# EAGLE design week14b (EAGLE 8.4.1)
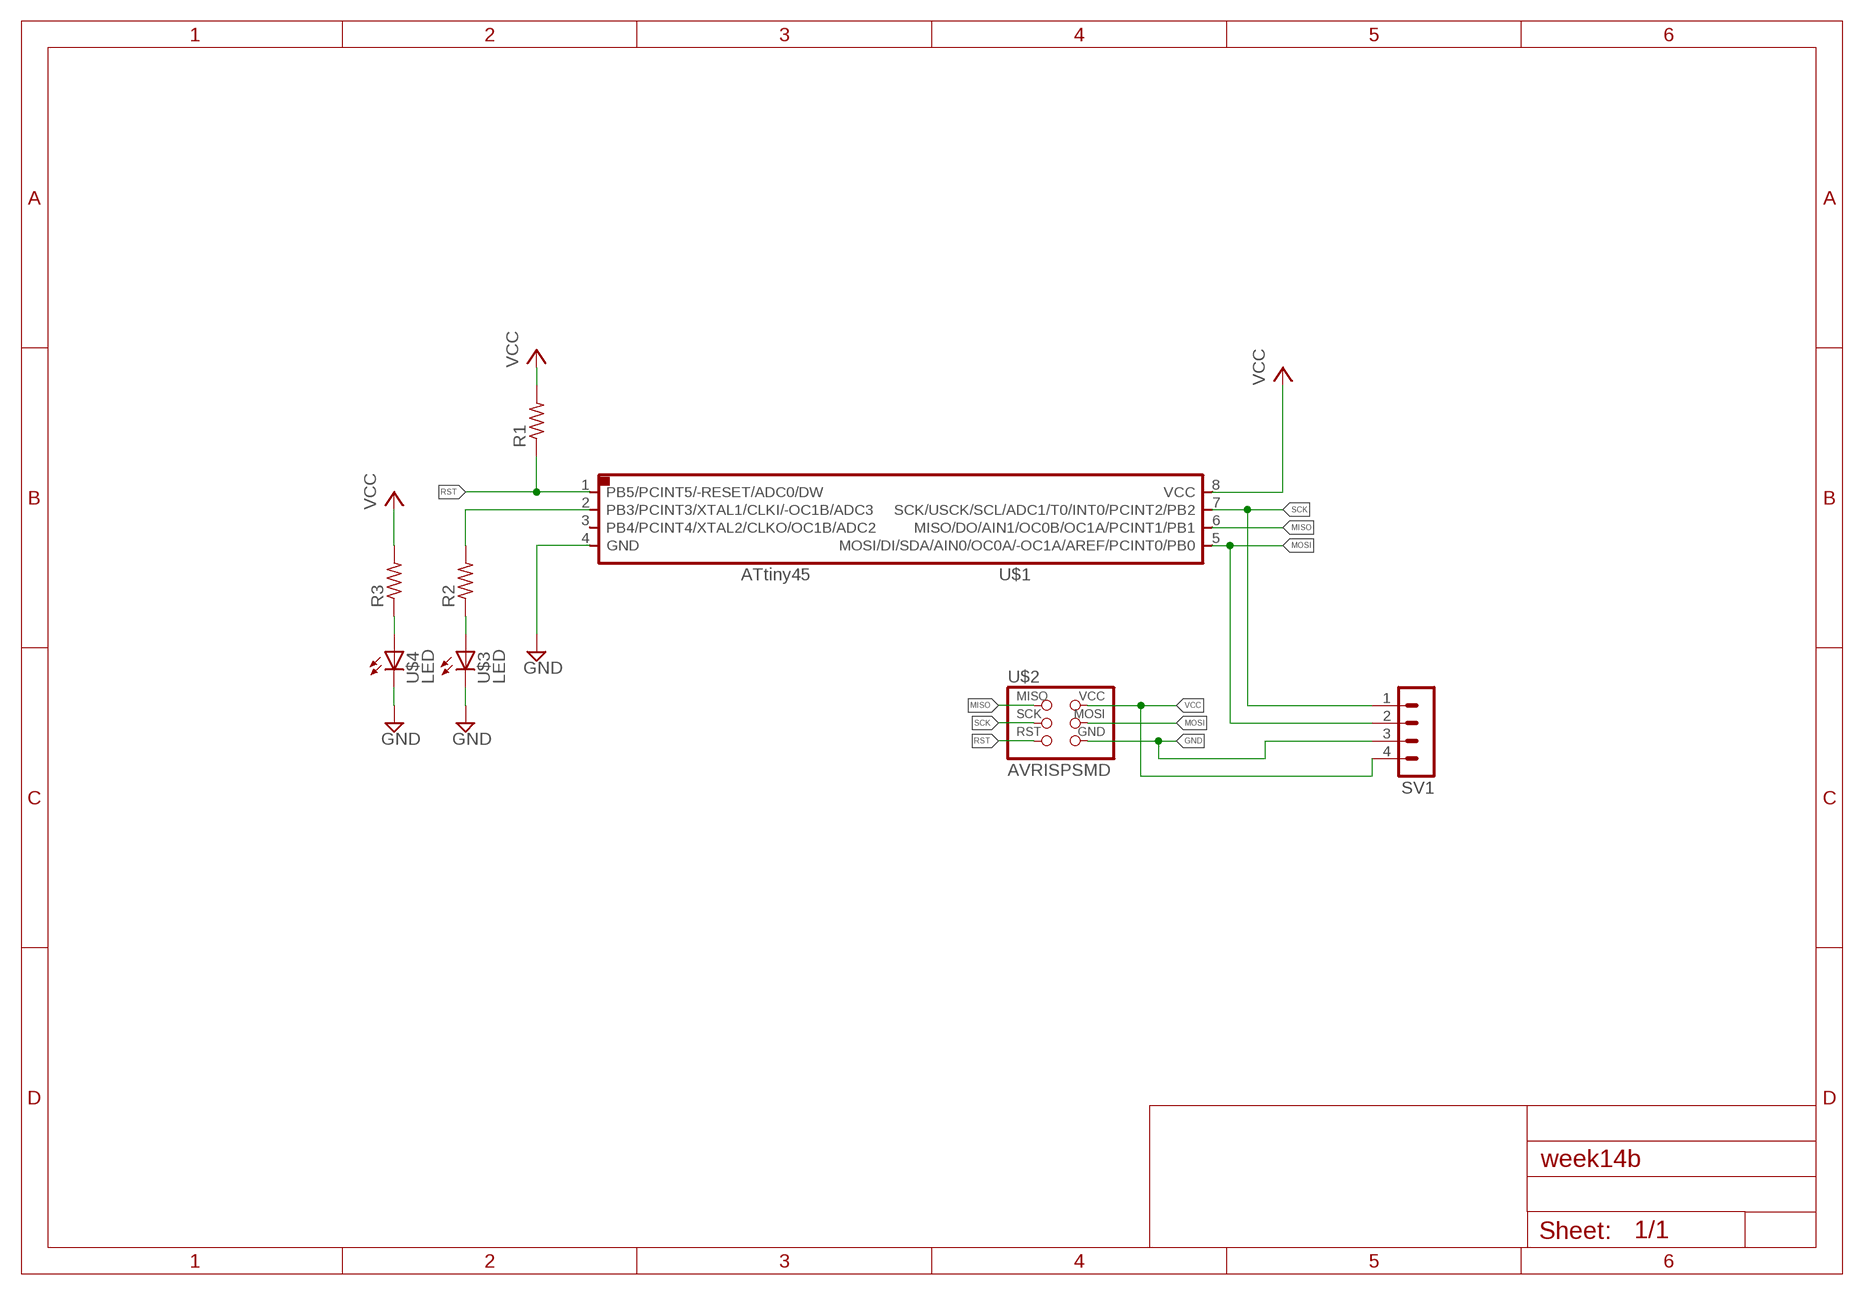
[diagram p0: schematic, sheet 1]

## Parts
R1  RES-US1206  [R1206]
R2  RES-US1206  [R1206]
R3  RES-US1206  [R1206]
SV1  MA04-1  [MA04-1]
U$1  ATTINY45SI  [SOIC8]
U$2  AVRISPSMD  [2X03SMD]
U$3  LED  [LED1206]
U$4  LED  [LED1206]

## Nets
GND: SV1.3 U$1.4(GND) U$2.6(GND) U$3.2(C) U$4.2(C)
MISO: U$1.6(MISO/DO/AIN1/OC0B/OC1A/PCINT1/PB1) U$2.1(MISO)
MOSI: SV1.2 U$1.5(MOSI/DI/SDA/AIN0/OC0A/-OC1A/AREF/PCINT0/PB0) U$2.4(MOSI)
N$2: R2.1 U$3.1(A)
N$3: R2.2 U$1.2(PB3/PCINT3/XTAL1/CLKI/-OC1B/ADC3)
N$5: R3.1 U$4.1(A)
RST: R1.1 U$1.1(PB5/PCINT5/-RESET/ADC0/DW) U$2.5(RST)
SCK: SV1.1 U$1.7(SCK/USCK/SCL/ADC1/T0/INT0/PCINT2/PB2) U$2.3(SCK)
VCC: R1.2 R3.2 SV1.4 U$1.8(VCC) U$2.2(VCC)
Unconnected: U$1.3(PB4/PCINT4/XTAL2/CLKO/OC1B/ADC2)

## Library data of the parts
R1-R3 = fab:RES-US: Resistor (US Symbol)
SV1 = con-lstb:MA04-1: PIN HEADER; OC_FARNELL: unknown; OC_NEWARK: unknown
U$1 = fab:ATTINY45
U$2 = fab:AVRISP
U$3 U$4 = fab:LED: LED

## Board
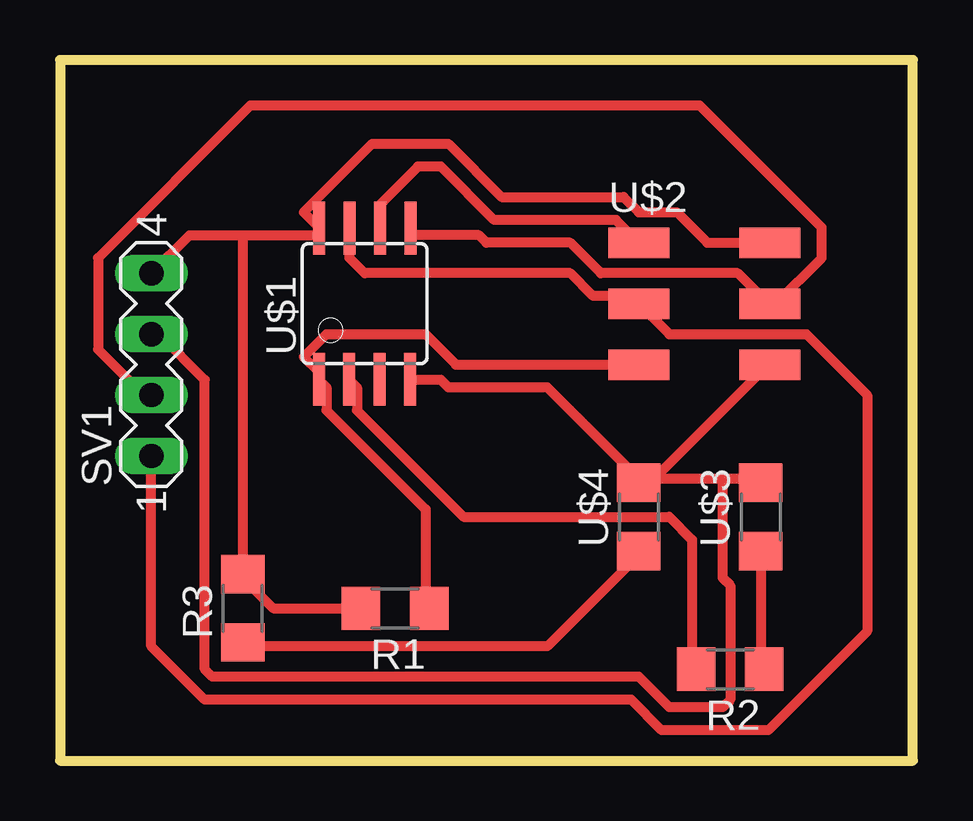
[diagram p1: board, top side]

Size 35.56 x 29.21 mm. Coordinates in mm from the lower left corner, seen from the top.
Outline: 0,29.21 0,0 35.56,0 35.56,29.21 0,29.21
Copper layers (1*16): Top 0.035mm / dielectric 1.5mm / Bottom 0.035mm
Design rules "default *": minimum track width 16mil, minimum drill 0.35mm, track to track 16mil, track to pad 16mil, pad to pad 16mil, via to via 6mil, smd to smd 16mil, copper to edge 16mil, drill to drill 16mil, minimum pad ring 10mil, minimum via ring 8mil, stop-mask expansion 4mil, vias tented up to drill 0mil, thermal gap 10mil

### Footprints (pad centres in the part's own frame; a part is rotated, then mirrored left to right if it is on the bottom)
R1206 = smd 1.6 x 1.803: 1 -1.422,0; 2 1.422,0
MA04-1 = drill 1.016 long: 1 -3.81,0; 2 -1.27,0; 3 1.27,0; 4 3.81,0
SOIC8 = smd 0.5 x 2.2: 1 -1.905,-3.154; 2 -0.645,-3.154; 3 0.625,-3.154; 4 1.895,-3.154; 5 1.905,3.154; 6 0.635,3.154; 7 -0.635,3.154; 8 -1.905,3.154
2X03SMD = smd 2.54 x 1.27: 1 -2.54,2.54; 2 2.92,2.54; 3 -2.54,0; 4 2.92,0; 5 -2.54,-2.54; 6 2.92,-2.54
LED1206 = smd 1.6 x 1.803: 1 -1.422,0; 2 1.422,0

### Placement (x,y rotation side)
R1  13.97,6.35 180 top
R2  27.94,3.81 180 top
R3  7.62,6.35 90 top
SV1  3.81,16.51 90 top
U$1  12.7,19.05 0 top
U$2  26.67,19.05 0 top
U$3  29.21,10.16 90 top
U$4  24.13,10.16 90 top

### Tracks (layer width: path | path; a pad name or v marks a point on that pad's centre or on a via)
GND
  Top 0.406: 27.62,11.75 29.21,11.75 U$3.2 | 27.62,11.75 24.77,11.75 | 24.77,11.75 24.13,11.75 | 24.13,11.75 20.32,15.56 16.19,15.56 15.87,15.88 14.6,15.88 U$1.4 | 24.13,11.75 U$4.2 24.77,11.75 | 24.77,11.75 29.53,16.51 U$2.6 | SV1.3 4.13,17.78 6.03,15.88 6.03,3.81 6.35,3.49 24.13,3.49 25.4,2.22 27.62,2.22 27.94,2.54 27.94,7.3 27.62,7.62 27.62,11.75
MISO
  Top 0.406: U$1.6 13.33,23.18 14.92,24.77 15.87,24.77 18.1,22.54 23.18,22.54 U$2.1
MOSI
  Top 0.406: U$1.5 14.6,21.91 17.46,21.91 17.78,21.59 21.27,21.59 22.54,20.32 28.26,20.32 29.53,19.05 U$2.4 29.84,19.05 31.75,20.95 31.75,22.23 26.67,27.3 7.94,27.3 1.59,20.95 1.59,17.15 3.49,15.24 SV1.2
N$2
  Top 0.406: U$3.1 29.21,3.81 R2.1
N$3
  Top 0.406: R2.2 26.35,3.81 26.35,9.21 25.4,10.16 16.83,10.16 12.38,14.6 12.38,15.56 12.06,15.88 U$1.2
N$5
  Top 0.406: R3.1 7.62,4.76 20.32,4.76 24.13,8.57 U$4.1
RST
  Top 0.406: R1.1 15.24,6.35 15.24,10.48 11.11,14.6 11.11,15.56 10.79,15.88 U$1.1 10.79,16.19 10.16,16.83 11.11,17.78 15.24,17.78 16.51,16.51 U$2.5
SCK
  Top 0.406: U$1.7 12.06,20.95 12.7,20.32 21.27,20.32 22.23,19.37 23.81,19.37 U$2.3 25.4,17.78 31.12,17.78 33.66,15.24 33.66,5.4 29.53,1.27 25.08,1.27 23.81,2.54 6.03,2.54 3.81,4.76 SV1.1
VCC
  Top 0.406: R1.2 8.89,6.35 7.62,7.62 R3.2 7.62,21.91 | 7.62,21.91 5.4,21.91 SV1.4 | 7.62,21.91 10.79,21.91 U$1.8 10.79,22.23 10.16,22.86 13.02,25.72 16.19,25.72 18.41,23.49 23.5,23.49 24.13,22.86 25.72,22.86 26.99,21.59 U$2.2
